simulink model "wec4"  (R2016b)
settings: Solver=ode4  StartTime=0  StopTime=1000  FixedStep=0.005  MaxStep=0.005  RelTol=1e-3  EnableMultiTasking=on
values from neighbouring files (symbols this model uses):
  arAdaptiveLawData = 1/2*zModelSimple.zModelPto.arFreq.*     zModelSimple.zModelPto.arMagnitude./     cos(zModelSimple.zModelPto.arPhase*pi/180+pi/2)    [IMPACT_Control.m]
  arAdaptiveLawDataX = 1/2*zModelSimpleX.zModelPto.arFreq.*         zModelSimpleX.zModelPto.arMagnitude./         cos(zModelSimpleX.zModelPto.arPhase*pi/180+pi/2)    [IMPACT_Control.m]
  arControllerRampGain = [0,0,1,1]    [IMPACT_Control.m]
  arControllerRampTime = [0 rStartRampTime rStartRampTime+rRampTimeLength 8000]    [IMPACT_Control.m]
  arEkfInitialisation = zeros(1,11)    [IMPACT_Control.m]
  arEkfInitialisationX = zeros(1,11)    [IMPACT_Control.m]
  arFrequency = zModelSimple.zModelPto.arFreq    [IMPACT_Control.m]
  arFrequencyRange = zModelSimple.zModelPto.arFreq    [IMPACT_Control.m]
  arFrequencyX = zModelSimpleX.zModelPto.arFreq    [IMPACT_Control.m]
  arImpedance = 1./zModelSimple.zModelPto.arMagnitude./zModelSimple.zModelPto.arFreq    [IMPACT_Control.m]
  arImpedanceX = 1./zModelSimpleX.zModelPto.arMagnitude./zModelSimpleX.zModelPto.arFreq    [IMPACT_Control.m]
  CentralPTOPreload = -1.6113e+07    (= -16113000)    [wecSimInputFile.m]
  F1 = [4.243 2.375 -12.243]    [wecSimInputFile.m]
  F2 = [4.243 -2.375 -12.243]    [wecSimInputFile.m]
  F3 = [-4.243 -2.375 -12.243]    [wecSimInputFile.m]
  F4 = [-4.243 2.375 -12.243]    [wecSimInputFile.m]
  FC = [0 0 -14]    [wecSimInputFile.m]
  iAdaptiveDamping = 0    [wec4IMPACT_Project.m]    (also in IMPACT_Control.m = handles.iAdaptiveDamping; wec1_IMPACT_Project.m; wec2_IMPACT_Project.m; wec3_IMPACT_Project.m)
  iControlType = 2    [wec4IMPACT_Project.m]    (also in IMPACT_Control.m = handles.iControlType; wec1_IMPACT_Project.m = 1; wec2_IMPACT_Project.m = 1; wec3_IMPACT_Project.m = 1)
  iPtoPositionConstraint = 1    [wec4IMPACT_Project.m]    (also in IMPACT_Control.m = handles.iPtoPositionConstraint; wec1_IMPACT_Project.m = 0; wec2_IMPACT_Project.m; wec3_IMPACT_Project.m)
  iSensorNoise = 0    [IMPACT_Control.m]
  m = m+1    (= 2)    [checkParamFile.m]
  PTOrotation = atan((T1(2)-F1(2))/(T1(1)-F1(1)))    [wecSimInputFile.m]
  rCogFloater = -8    [wec4_IMPACT_Model.m]    (also in paramInitial.m = get( handles.edit_rCogFloater, 'String' ); wec1_IMPACT_Model.m = -18; wec2_IMPACT_Model.m = -8.5; wec3_IMPACT_Model.m = -0.7)
  rCogSpar = -36.6    [wec4_IMPACT_Model.m]    (also in paramInitial.m = get( handles.edit_rCogSpar, 'String' ); wec3_IMPACT_Model.m = -21.3; wec3_IMPACT_Model2.m = -21.3)
  rDisplacementLimit = 10.000000    (= 10)    [wec4IMPACT_Project.m]    (also in IMPACT_Control.m = getValue(handles.edit_displacementLimit); wec1_IMPACT_Project.m; wec2_IMPACT_Project.m; wec3_IMPACT_Project.m = 3)
  rDisplacementLimitX = 10.000000    (= 10)    [wec4IMPACT_Project.m]    (also in IMPACT_Control.m = getValue(handles.edit_displacementLimitX); wec1_IMPACT_Project.m = 0; wec2_IMPACT_Project.m; wec3_IMPACT_Project.m = 0)
  rGainForAntiWIndUp = tfControllerDiscrete.rGain    [IMPACT_Control.m]
  rGainForAntiWIndUpX = tfControllerXDiscrete.rGain    [IMPACT_Control.m]
  rMaxForcePto = 300000000.000000    (= 300000000)    [wec4IMPACT_Project.m]    (also in IMPACT_Control.m = getValue(handles.edit_maxForcePto); wec1_IMPACT_Project.m = 1e+15; wec2_IMPACT_Project.m = 1e+15; wec3_IMPACT_Project.m = 1000000000)
  rMinForcePto = -300000000.000000    (= -300000000)    [wec4IMPACT_Project.m]    (also in IMPACT_Control.m = getValue(handles.edit_minForcePto); wec1_IMPACT_Project.m = -1e+15; wec2_IMPACT_Project.m = -1e+15; wec3_IMPACT_Project.m = -1000000000)
  rMooringX = 20000    [wec4_IMPACT_Model.m]    (also in paramInitial.m = get( handles.edit_rMooringX, 'String' ); wec3_IMPACT_Model.m = 10000; wec3_IMPACT_Model2.m = 10000)
  rMooringZ = 10000    [wec4_IMPACT_Model.m]    (also in paramInitial.m = get( handles.edit_rMooringZ, 'String' ); wec3_IMPACT_Model.m = 0; wec3_IMPACT_Model2.m = 0)
  rOutputSampleTime = 0.010000    (= 0.01)    [wec4IMPACT_Project.m]    (also in IMPACT_Control.m = getValue(handles.edit_outputSampleTime); wec1_IMPACT_Project.m; wec2_IMPACT_Project.m; wec3_IMPACT_Project.m)
  rPassiveDampingGain = -604830.000000    (= -604830)    [wec4IMPACT_Project.m]    (also in IMPACT_Control.m = getValue(handles.edit_gainPLD); wec1_IMPACT_Project.m = -214018.1537; wec2_IMPACT_Project.m = -1948070; wec3_IMPACT_Project.m = -519390)
  rPassiveDampingGainX = -278660.000000    (= -278660)    [wec4IMPACT_Project.m]    (also in IMPACT_Control.m = getValue(handles.edit_gainPLDX); wec1_IMPACT_Project.m = 0; wec2_IMPACT_Project.m = 0; wec3_IMPACT_Project.m = 0)
  rTetherPretension = 1.6113e+07    (= 16113000)    [wec4_IMPACT_Model.m]    (also in paramInitial.m = get( handles.edit_rTetherPretension, 'String' ); wec3_IMPACT_Model.m = 0; wec3_IMPACT_Model2.m = 0)
  rTetherSpring = 500000    [wec4_IMPACT_Model.m]    (also in paramInitial.m = get( handles.edit_rTetherSpring, 'String' ); wec3_IMPACT_Model.m = 0; wec3_IMPACT_Model2.m = 0)
  rUpperFrequencyLimit = EKFFloater.upperFreq    [IMPACT_Control.m]
  rXf = 4.243    [wec4AdditionalParams.m]
  rXs = 16.075    [wec4AdditionalParams.m]
  rYf = 2.375    [wec4AdditionalParams.m]
  rYs = 16.075    [wec4AdditionalParams.m]
  rZf = 4.243    [wec4AdditionalParams.m]
  rZs = 2.4350    (= 2.435)    [wec4AdditionalParams.m]
  rZTetherF = 6    [wec4AdditionalParams.m]
  rZTetherS = 2.4350    (= 2.435)    [wec4AdditionalParams.m]
  s = tf('s')    [wec4_IMPACT_Model.m]    (also in IMPACT_Control.m; wec1_IMPACT_Model.m; wec2_IMPACT_Model.m; wec3_IMPACT_Model.m)
  SidePTO1Preload = PreloadPTOCorner    (= 0)    [wecSimInputFile.m]
  SidePTO2Preload = PreloadPTOCorner    (= 0)    [wecSimInputFile.m]
  SidePTO3Preload = PreloadPTOCorner    (= 0)    [wecSimInputFile.m]
  SidePTO4Preload = PreloadPTOCorner    (= 0)    [wecSimInputFile.m]
  simu = simulationClass()    [wecSimInputFile.m]
  T1 = [16.075 16.075 -34.165]    [wecSimInputFile.m]
  T2 = [16.075 -16.075 -34.165]    [wecSimInputFile.m]
  T3 = [-16.075 -16.075 -34.165]    [wecSimInputFile.m]
  T4 = [-16.075 16.075 -34.165]    [wecSimInputFile.m]
  TC = [0 0 -34.165]    [wecSimInputFile.m]
  waves = waveClass('irregular')    [wecSimInputFile.m]
  Z = magPhaseToComplex(zModelTf)    [IMPACT_Control.m]
undefined symbols (not defined in the file or in its folder): arControllerDiscreteDen, arControllerDiscreteNum, arControllerDiscreteXDen, arControllerDiscreteXNum, arExcForceFloaterDen, arExcForceFloaterNum, arExcForceFloaterXDen, arExcForceFloaterXNum, arExcForceSparDen, arExcForceSparNum, arExcForceSparXDen, arExcForceSparXNum, arFexcFloaterDen, arFexcFloaterNum, arFexcFloaterXDen, arFexcFloaterXNum, arFexcSparDen, arFexcSparNum, arFexcSparXDen, arFexcSparXNum, Body, body, constraint, CTTime, deg, Elements, geometry, IRKB, kg, lenJ, mooring, N, pto, rAccelerationGainFloater, rAccelerationGainFloaterX, rAccelerationGainSpar, rAccelerationGainSparX, rad, rBuoyancyGainFloater, rBuoyancyGainFloaterX, rBuoyancyGainSpar, rBuoyancyGainSparX, rDampingGainFloater, rDampingGainFloaterX, rDampingGainSpar, rDampingGainSparX, Rigid, rMaxFocePto, wec4_float, wec4_reactor, WECSim_Lib, X, Y
libraries: nesl_utility x380, sm_lib x170, vrlib x91, simulink x12, WECSim_Lib x4
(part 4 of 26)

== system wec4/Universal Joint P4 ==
  Assignment : Assignment  DiagnosticForDimensions=Warning  IndexOptions=Index vector (dialog)  Indices=[4 5]  OutputSizes=1
  Assignment1 : Assignment  DiagnosticForDimensions=Warning  IndexOptions=Index vector (dialog)  Indices=[4 5]  OutputSizes=1
  Assignment2 : Assignment  DiagnosticForDimensions=Warning  IndexOptions=Index vector (dialog)  Indices=[4 5]  OutputSizes=1
  CONSTRAINT Universal Joint : sm_lib/Joints/Universal Joint  SenseConstraintForce=on  SenseConstraintForceX=off  SenseConstraintForceY=off  SenseConstraintForceZ=off  SenseConstraintTorque=on  SenseConstraintTorqueX=off  SenseConstraintTorqueY=off  SenseConstraintTorqueZ=off  SenseTotalForce=off  SenseTotalForceX=off  SenseTotalForceY=off  SenseTotalForceZ=off  SenseTotalTorque=off  SenseTotalTorqueX=off  SenseTotalTorqueY=off  SenseTotalTorqueZ=off  CompositeWrenchDir=BaseOnFollower  CompositeWrenchFrame=BaseFrame  RxEquilibriumPosition=0  RxEquilibriumPositionUnits=deg  RxSpringStiffness=0  RxSpringStiffnessUnits=N*m/deg  RxDampingCoefficient=0  RxDampingCoefficientUnits=N*m/(deg/s)  RxTorqueActuationMode=NoTorque  RxMotionActuationMode=ComputedMotion  RxSensePosition=on  RxSenseVelocity=on  RxSenseAcceleration=on  RxSenseTorqueForce=off  RxPositionTargetSpecify=off  RxPositionTargetPriority=High  RxPositionTargetValue=0  RxPositionTargetValueUnits=deg  RxVelocityTargetSpecify=off  RxVelocityTargetPriority=High  RxVelocityTargetValue=0  RxVelocityTargetValueUnits=deg/s  RyEquilibriumPosition=0  RyEquilibriumPositionUnits=deg  RySpringStiffness=0  RySpringStiffnessUnits=N*m/deg  RyDampingCoefficient=0  RyDampingCoefficientUnits=N*m/(deg/s)  RyTorqueActuationMode=NoTorque  RyMotionActuationMode=ComputedMotion  RySensePosition=on  RySenseVelocity=on  RySenseAcceleration=on  RySenseTorqueForce=off  RyPositionTargetSpecify=off  RyPositionTargetPriority=High  RyPositionTargetValue=0  RyPositionTargetValueUnits=deg  RyVelocityTargetSpecify=off  RyVelocityTargetPriority=High  RyVelocityTargetValue=0  RyVelocityTargetValueUnits=deg/s
  Constant : Constant  Value=[0 0 0 0 0 0]
  Constant1 : Constant  Value=[0 0 0 0 0 0]
  Constant2 : Constant  Value=[0 0 0 0 0 0]
  Mux{,2..4} (4 alike) : Mux  Inputs=2
  Mux1 : Mux
  PS-Simulink Converter{1..5,7,9,11} (8 alike) : nesl_utility/PS-Simulink Converter  PhysicalDomain=network_engine_domain  SubClassName=ps_output  LeftPortType=input  RightPortType=output  PseudoPeriodic=off  Frequencies=[]  Unit=1  AffineConversion=off
  Rigid Transform (Position) : sm_lib/Frames and Transforms/Rigid Transform  TranslationMethod=Cartesian  TranslationStandardOffset=0  TranslationLengthUnit=m  TranslationStandardAxis=+Z  TranslationCartesianOffset=constraint.initDisp.initLinDisp+constraint.loc  TranslationROffset=0  TranslationROffsetUnits=m  TranslationZOffset=0  TranslationZOffsetUnits=m  TranslationThetaOffset=0  TranslationThetaOffsetUnits=deg  RotationMethod=None  RotationAngleUnits=rad  RotationStandardAxis=+Y  RotationAngle=0  RotationArbitraryAxis=[0 1 0]  FollAlignAxisA=+X  BaseAlignAxisA=+Y  FollAlignAxisB=+Y  BaseAlignAxisB=+Z  RotationSequenceAxes=FollowerAxes  RotationSequence=XYX  RotationSequenceAngles=[0 0 0]  RotationSequenceAnglesUnits=deg  RotationMatrix=[1 0 0; 0 1 0; 0 0 1]
  Rigid Transform (Position)1 : sm_lib/Frames and Transforms/Rigid Transform  TranslationMethod=Cartesian  TranslationStandardOffset=0  TranslationLengthUnit=m  TranslationStandardAxis=+Z  TranslationCartesianOffset=constraint.initDisp.initLinDisp+constraint.loc  TranslationROffset=0  TranslationROffsetUnits=m  TranslationZOffset=0  TranslationZOffsetUnits=m  TranslationThetaOffset=0  TranslationThetaOffsetUnits=deg  RotationMethod=None  RotationAngleUnits=rad  RotationStandardAxis=+Y  RotationAngle=0  RotationArbitraryAxis=[0 1 0]  FollAlignAxisA=+X  BaseAlignAxisA=+Y  FollAlignAxisB=+Y  BaseAlignAxisB=+Z  RotationSequenceAxes=FollowerAxes  RotationSequence=XYX  RotationSequenceAngles=[0 0 0]  RotationSequenceAnglesUnits=deg  RotationMatrix=[1 0 0; 0 1 0; 0 0 1]
  Rigid Transform (Orientation) : sm_lib/Frames and Transforms/Rigid Transform  TranslationMethod=None  TranslationStandardOffset=0  TranslationLengthUnit=m  TranslationStandardAxis=+Z  TranslationCartesianOffset=constraint.loc  TranslationROffset=0  TranslationROffsetUnits=m  TranslationZOffset=0  TranslationZOffsetUnits=m  TranslationThetaOffset=0  TranslationThetaOffsetUnits=deg  RotationMethod=RotationMatrix  RotationAngleUnits=rad  RotationStandardAxis=+Y  RotationAngle=0  RotationArbitraryAxis=[0 1 0]  FollAlignAxisA=+X  BaseAlignAxisA=+Y  FollAlignAxisB=+Y  BaseAlignAxisB=+Z  RotationSequenceAxes=FollowerAxes  RotationSequence=XYX  RotationSequenceAngles=[0 0 0]  RotationSequenceAnglesUnits=deg  RotationMatrix=constraint.orientation.rotationMatrix
  Rigid Transform (Orientation)1 : sm_lib/Frames and Transforms/Rigid Transform  TranslationMethod=None  TranslationStandardOffset=0  TranslationLengthUnit=m  TranslationStandardAxis=+Z  TranslationCartesianOffset=constraint.loc  TranslationROffset=0  TranslationROffsetUnits=m  TranslationZOffset=0  TranslationZOffsetUnits=m  TranslationThetaOffset=0  TranslationThetaOffsetUnits=deg  RotationMethod=RotationMatrix  RotationAngleUnits=rad  RotationStandardAxis=+Y  RotationAngle=0  RotationArbitraryAxis=[0 1 0]  FollAlignAxisA=+X  BaseAlignAxisA=+Y  FollAlignAxisB=+Y  BaseAlignAxisB=+Z  RotationSequenceAxes=FollowerAxes  RotationSequence=XYX  RotationSequenceAngles=[0 0 0]  RotationSequenceAnglesUnits=deg  RotationMatrix=constraint.orientation.rotationMatrix
  output : ToWorkspace  VariableName=constraint10_out  SaveFormat=Structure With Time  SampleTime=-1
  F : PMIOPort  Port=1  Side=Right
  B : PMIOPort  Port=2  Side=Left
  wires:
  PS-Simulink Converter4/1 -> Mux/2
  PS-Simulink Converter3/1 -> Mux/1
  Mux3/1 -> Assignment1/2
  Mux4/1 -> Assignment/2
  Constant/1 -> Assignment/1
  Constant1/1 -> Assignment1/1
  Constant2/1 -> Assignment2/1
  Assignment2/1 -> Mux1/3  "acceleration"
  Assignment1/1 -> Mux1/2  "velocity"
  Assignment/1 -> Mux1/1  "position"
  Mux/1 -> Mux1/4  "Constraint Forces"
  Mux1/1 -> output/1
  PS-Simulink Converter5/1 -> Mux2/2
  Mux2/1 -> Assignment2/2
  PS-Simulink Converter2/1 -> Mux3/2
  PS-Simulink Converter9/1 -> Mux3/1
  PS-Simulink Converter11/1 -> Mux4/2
  PS-Simulink Converter1/1 -> Mux4/1
  PS-Simulink Converter7/1 -> Mux2/1
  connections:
  Rigid Transform (Position)1/LConn1 -- F/RConn1
  Rigid Transform (Position)1/RConn1 -- Rigid Transform (Orientation)1/LConn1
  Rigid Transform (Orientation)/RConn1 -- CONSTRAINT Universal Joint/LConn1
  Rigid Transform (Position)/RConn1 -- Rigid Transform (Orientation)/LConn1
  Rigid Transform (Position)/LConn1 -- B/RConn1
  CONSTRAINT Universal Joint/RConn8 -- PS-Simulink Converter3/LConn1
  PS-Simulink Converter4/LConn1 -- CONSTRAINT Universal Joint/RConn9
  PS-Simulink Converter1/LConn1 -- CONSTRAINT Universal Joint/RConn2
  PS-Simulink Converter11/LConn1 -- CONSTRAINT Universal Joint/RConn5
  PS-Simulink Converter9/LConn1 -- CONSTRAINT Universal Joint/RConn3
  PS-Simulink Converter7/LConn1 -- CONSTRAINT Universal Joint/RConn4
  PS-Simulink Converter2/LConn1 -- CONSTRAINT Universal Joint/RConn6
  PS-Simulink Converter5/LConn1 -- CONSTRAINT Universal Joint/RConn7
  CONSTRAINT Universal Joint/RConn1 -- Rigid Transform (Orientation)1/RConn1

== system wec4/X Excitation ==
  PTO force X : Inport
  Force estimation Floater X : Subsystem
  Force estimation Spar X : Subsystem
  Gain12 : Gain  Gain=rMooringX
  Gain3 : Gain  Gain=-1
  Rate Transition3 : RateTransition  OutPortSampleTimeMultiple=0.01  OutPortSampleTime=rKalmanFilterSampleTime
  Rate Transition4 : RateTransition  OutPortSampleTimeMultiple=0.01  OutPortSampleTime=rKalmanFilterSampleTime
  Scope{11..14} (4 alike) : Scope
  Selector{7..12,22} (7 alike) : Selector  InputPortWidth=6  IndexOptions=Index vector (dialog)  Indices=1  OutputSizes=1
  Sum11 : Sum
  Sum4 : Sum  Inputs=|++
  Sum5 : Sum  Inputs=|+-
  To Workspace11 : ToWorkspace  VariableName=arForceXFloater  SampleTime=rOutputSampleTime
  To Workspace5 : ToWorkspace  VariableName=arExcitationForceSparX  SampleTime=rOutputSampleTime
  To Workspace6 : ToWorkspace  VariableName=arExcitationForceFloaterX  SampleTime=rOutputSampleTime
  floaterExcitation : Outport
  SparExcitation : Outport  Port=2
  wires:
  Sum4/1 -> Scope14/1
  Selector8/1 -> Force estimation Floater X/3(Position)
  Selector7/1 -> Force estimation Floater X/2(Velocity)
  [acc1] -> Selector9/1
  [acc2] -> Selector12/1
  Sum5/1 -> Scope11/1
  Gain3/1 -> Sum11/1
  [vel1] -> Selector7/1
  Selector10/1 -> Force estimation Spar X/2(Velocity)
  [disp1] -> Selector8/1
  Selector12/1 -> Force estimation Spar X/1(Acceleration)
  Selector11/1 -> Force estimation Spar X/3(Position)
  Selector9/1 -> Force estimation Floater X/1(Acceleration)
  Force estimation Spar X/1(excForce) -> Rate Transition4/1
  Rate Transition3/1 -> To Workspace6/1, floaterExcitation/1, Scope13/1, Sum4/1, Sum5/1
  [disp2] -> Selector11/1
  Force estimation Floater X/1(excForce) -> Rate Transition3/1
  [vel2] -> Selector10/1
  PTO force X/1 -> Force estimation Floater X/4(PTO Force), Gain3/1, To Workspace11/1
  [disp2] -> Selector22/1
  Selector22/1 -> Gain12/1
  Gain12/1 -> Sum11/2
  Sum11/1 -> Force estimation Spar X/4(PTO Force)
  Rate Transition4/1 -> To Workspace5/1, SparExcitation/1, Sum4/2, Sum5/2, Scope12/1

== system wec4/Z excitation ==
  PTO force Z : Inport
  Constant2 : Constant  Value=rCogSpar
  "Force estimation Floater " : Subsystem
  Force estimation Spar : Subsystem
  Gain : Gain  Gain=-1
  Gain12 : Gain  Gain=rMooringZ
  Rate Transition1 : RateTransition  OutPortSampleTimeMultiple=0.01  OutPortSampleTime=rKalmanFilterSampleTime
  Rate Transition2 : RateTransition  OutPortSampleTimeMultiple=0.01  OutPortSampleTime=rKalmanFilterSampleTime
  Selector{1..6,22} (7 alike) : Selector  InputPortWidth=6  IndexOptions=Index vector (dialog)  Indices=3  OutputSizes=1
  Sum11 : Sum
  Sum20 : Sum  Inputs=+-
  To Workspace4 : ToWorkspace  VariableName=arExcitationForceSpar  SampleTime=rOutputSampleTime
  To Workspace7 : ToWorkspace  VariableName=arExcitationForceFloater  SampleTime=rOutputSampleTime
  floaterExcitation : Outport
  SparExcitation : Outport  Port=2
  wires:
  Selector4/1 -> Force estimation Spar/2(Velocity)
  Rate Transition2/1 -> SparExcitation/1, To Workspace4/1
  Selector5/1 -> Force estimation Spar/3(Position)
  Gain/1 -> Sum11/1
  "Force estimation Floater "/1(excForce) -> Rate Transition1/1
  [acc1] -> Selector3/1
  Force estimation Spar/1(excForce) -> Rate Transition2/1
  [vel1] -> Selector1/1
  Rate Transition1/1 -> floaterExcitation/1, To Workspace7/1
  PTO force Z/1 -> "Force estimation Floater "/4(PTO Force), Gain/1
  Selector6/1 -> Force estimation Spar/1(Acceleration)
  [acc2] -> Selector6/1
  [vel2] -> Selector4/1
  [disp1] -> Selector2/1
  [disp2] -> Selector5/1
  Constant2/1 -> Sum20/2
  [disp2] -> Selector22/1
  Gain12/1 -> Sum11/2
  Sum20/1 -> Gain12/1
  Sum11/1 -> Force estimation Spar/4(PTO Force)
  Selector22/1 -> Sum20/1
  Selector3/1 -> "Force estimation Floater "/1(Acceleration)
  Selector1/1 -> "Force estimation Floater "/2(Velocity)
  Selector2/1 -> "Force estimation Floater "/3(Position)

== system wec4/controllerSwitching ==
  ovtForceDemand1 : Inport
  ovtForceDemand2 : Inport  Port=2
  ovtForceDemand3 : Inport  Port=3
  ovtForceDemand4 : Inport  Port=4
  linearDampingForce1 : Inport  Port=5
  linearDampingForce2 : Inport  Port=6
  linearDampingForce3 : Inport  Port=7
  linearDampingForce4 : Inport  Port=8
  Constant2 : Constant  Value=iControlType
  Mux1 : Mux
  Mux11 : Mux
  Saturation : Saturate  Commented=through  UpperLimit=rMaxForcePto  LowerLimit=-rMaxFocePto
  Switch1 : Switch  Threshold=2
  forceDemand : Outport
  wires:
  linearDampingForce1/1 -> Mux1/1
  linearDampingForce2/1 -> Mux1/2
  linearDampingForce3/1 -> Mux1/3
  linearDampingForce4/1 -> Mux1/4
  Constant2/1 -> Switch1/2
  Mux11/1 -> Switch1/3
  Mux1/1 -> Switch1/1
  Switch1/1 -> Saturation/1
  Saturation/1 -> forceDemand/1
  ovtForceDemand1/1 -> Mux11/1
  ovtForceDemand2/1 -> Mux11/2
  ovtForceDemand3/1 -> Mux11/3
  ovtForceDemand4/1 -> Mux11/4

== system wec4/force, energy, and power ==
  Gain1 : Gain  Gain=-1
  Integrator : Integrator
  Mux1 : Mux
  Product{,1..3} (4 alike) : Product
  Scope : Scope
  Scope6 : Scope
  Scope7 : Scope
  Sum : Sum  Inputs=++++
  To Workspace1 : ToWorkspace  VariableName=arPtoForceOutput  SampleTime=rOutputSampleTime
  To Workspace2 : ToWorkspace  VariableName=arWecPower  SampleTime=rOutputSampleTime
  To Workspace3 : ToWorkspace  VariableName=arWecEnergy  SampleTime=rOutputSampleTime
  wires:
  Mux1/1 -> To Workspace1/1, Scope/1
  [ptoForce4] -> Product3/2, Mux1/4
  [ptoForce3] -> Product2/1, Mux1/3
  [ptoForce2] -> Product1/1, Mux1/2
  [ptoForce1] -> Product/1, Mux1/1
  [ptoSpd1] -> Product/2
  [ptoSpd2] -> Product1/2
  [ptoSpd3] -> Product2/2
  [ptoSpd4] -> Product3/1
  Product/1 -> Sum/1
  Product1/1 -> Sum/2
  Product2/1 -> Sum/3
  Product3/1 -> Sum/4
  Sum/1 -> Gain1/1
  Integrator/1 -> Scope6/1, To Workspace3/1
  Gain1/1 -> Integrator/1, Scope7/1, To Workspace2/1

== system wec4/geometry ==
  Constant : Constant  Value="sqrt( (F1(1)-T1(1))^2 + (F1(2)-T1(2))^2 + (F1(3)-T1(3))^2  )"
  Demux{1..3,8} (4 alike) : Demux
  Divide : Product  Inputs=/*
  Geometry1 : Subsystem
  Math Function : Math  Operator=square
  Math Function1 : Math  Operator=square
  Mux{1,12,14,24} (4 alike) : Mux
  Sqrt : Sqrt
  Subsystem4 : Subsystem
  Sum : Sum  Inputs=|++
  Sum1 : Sum  Inputs=|++
  "Terminator2 " : Terminator
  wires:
  Demux8/4 -> [kappa4]
  Demux2/1 -> [beta1]
  Demux2/3 -> [beta3]
  Demux3/3 -> [gamma3]
  Demux8/1 -> [kappa1]
  Demux8/3 -> [kappa3]
  Mux12/1 -> Subsystem4/2(mus)
  Mux14/1 -> [zetas], Math Function/1, Subsystem4/1(Zetas)
  Geometry1/1(zeta1) -> Mux14/1
  Geometry1/2(zeta2) -> Mux14/2
  Geometry1/3(zeta3) -> Mux14/3
  Geometry1/4(zeta4) -> Mux14/4
  Geometry1/5(mu1) -> Mux12/1
  Geometry1/6(mu2) -> Mux12/2
  Geometry1/7(mu3) -> Mux12/3
  Geometry1/8(mu4) -> Mux12/4
  Mux24/1 -> Math Function1/1, Subsystem4/3(etas), [etas]
  Geometry1/9(eta1) -> Mux24/1
  Geometry1/10(eta2) -> Mux24/2
  Geometry1/11(eta3) -> Mux24/3
  Geometry1/12(eta4) -> Mux24/4
  Demux3/1 -> [gamma1]
  Demux3/4 -> [gamma4]
  Subsystem4/2(betas) -> Demux2/1
  Demux2/4 -> [beta4]
  Demux2/2 -> [beta2]
  Demux3/2 -> [gamma2]
  Demux8/2 -> [kappa2]
  Subsystem4/4(alphas) -> Demux8/1
  Math Function/1 -> Sum/1
  Math Function1/1 -> Sum/2
  Sum/1 -> Sqrt/1
  [ptoDis1] -> Mux1/1
  [ptoDis2] -> Mux1/2
  [ptoDis3] -> Mux1/3
  [ptoDis4] -> Mux1/4
  Mux1/1 -> Sum1/2
  Sqrt/1 -> Divide/2
  Divide/1 -> Demux1/1
  Constant/1 -> Sum1/1
  Sum1/1 -> Divide/1
  Demux1/1 -> [cosAlpha1]
  Demux1/2 -> [cosAlpha2]
  Demux1/3 -> [cosAlpha3]
  Demux1/4 -> [cosAlpha4]
  Subsystem4/3(deltas) -> "Terminator2 "/1
  Subsystem4/1(gammas) -> Demux3/1

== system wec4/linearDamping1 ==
  ekfFrequencyZ : Inport
  ekfFrequencyX : Inport  Port=2
  Rel. vel X : Inport  Port=3
  Rel. vel. Z : Inport  Port=4
  Clock1 : Clock
  Constant3 : Constant  Value=iAdaptiveDamping
  Constant4 : Constant  Value=rPassiveDampingGain
  Constant5 : Constant  Value=iAdaptiveDamping
  Constant6 : Constant  Value=rPassiveDampingGainX
  Gain1 : Gain  Gain=-1
  Gain3 : Gain  Gain=-1
  Product{1..3,11} (4 alike) : Product
  Ramp gain2 : Lookup_n-D  NumberOfTableDimensions=1  BreakpointsForDimension1=arControllerRampTime  Table=arControllerRampGain  InternalRulePriority=Speed  RndMeth=Simplest
  Switch1 : Switch  Criteria=u2 > Threshold
  Switch2 : Switch  Criteria=u2 > Threshold
  Trnasformation X-Z into PTO forces : Subsystem
  adaptiveLaw1 : Lookup_n-D  NumberOfTableDimensions=1  BreakpointsForDimension1=arFrequencyX  Table=arImpedanceX  InternalRulePriority=Speed  RndMeth=Simplest
  adaptiveLaw2 : Lookup_n-D  NumberOfTableDimensions=1  BreakpointsForDimension1=arFrequency  Table=arImpedance  InternalRulePriority=Speed  RndMeth=Simplest
  forceDemand1 : Outport
  forceDemand2 : Outport  Port=2
  forceDemand3 : Outport  Port=3
  forceDemand4 : Outport  Port=4
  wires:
  adaptiveLaw2/1 -> Gain3/1
  ekfFrequencyZ/1 -> adaptiveLaw2/1
  adaptiveLaw1/1 -> Gain1/1
  ekfFrequencyX/1 -> adaptiveLaw1/1
  Constant3/1 -> Switch2/2
  Gain3/1 -> Switch2/1  "K_z"
  Constant4/1 -> Switch2/3
  Constant5/1 -> Switch1/2
  Gain1/1 -> Switch1/1  "K_x"
  Constant6/1 -> Switch1/3
  Switch2/1 -> Product2/1  "Impedance Z"
  Switch1/1 -> Product1/2  "Impedance X"
  Clock1/1 -> Ramp gain2/1
  Ramp gain2/1 -> Product3/1, Product11/2
  Product3/1 -> forceDemand2/1, forceDemand1/1  "F1"
  Trnasformation X-Z into PTO forces/1(Force PTOs 3-4) -> Product11/1
  Product11/1 -> forceDemand4/1, forceDemand3/1
  Trnasformation X-Z into PTO forces/2(Force PTOs 1-2) -> Product3/2
  Rel. vel. Z/1 -> Product2/2
  Rel. vel X/1 -> Product1/1
  Product1/1 -> Trnasformation X-Z into PTO forces/1(Force X)
  Product2/1 -> Trnasformation X-Z into PTO forces/2(Force Z)

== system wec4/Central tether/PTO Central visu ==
  note: 1) Add Subsystem or Model blocks as valid variant choices. 2) You cannot connect blocks at this level. At simulation, connectivity is automatically determined, based on the active variant and port name matching.
  Hydrodynamic Body : Subsystem  VariantControl=sv_b3_hydroBody
  Non-Hydro Body : Subsystem  VariantControl=sv_b3_nonHydroBody
  Conn : PMIOPort  Port=1  Side=Right

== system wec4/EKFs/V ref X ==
  phiOut : Inport
  ekfFrequency : Inport  Port=2
  ekfAmplitude : Inport  Port=3
  Constraint : Subsystem
  Divide4 : Product  Inputs=**
  Gain1 : Gain
  Product1 : Product
  Scope2 : Scope
  Transfer Fcn : TransferFcn  Denominator=[0.05 1]
  adaptiveLaw : Lookup_n-D  NumberOfTableDimensions=1  BreakpointsForDimension1=arFrequencyRange  Table=arAdaptiveLawDataX  InternalRulePriority=Speed  RndMeth=Simplest
  adaptiveLaw1 : Lookup_n-D  NumberOfTableDimensions=1  BreakpointsForDimension1=arFrequencyRange  Table=arFrequencyRange./arFrequencyRange  InternalRulePriority=Speed  RndMeth=Simplest
  referenceVelocity : Outport
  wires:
  Transfer Fcn/1 -> Product1/2
  Product1/1 -> Scope2/1, Divide4/1
  ekfAmplitude/1 -> Constraint/2(Amp)
  phiOut/1 -> Transfer Fcn/1
  ekfFrequency/1 -> adaptiveLaw/1, adaptiveLaw1/1, Constraint/3(ekfFrequency)
  Divide4/1 -> referenceVelocity/1
  adaptiveLaw/1 -> Gain1/1
  Gain1/1 -> Constraint/1(1/2B)
  Constraint/1(referenceVelocity) -> Product1/1
  adaptiveLaw1/1 -> Divide4/2

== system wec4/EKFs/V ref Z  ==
  phiOut : Inport
  ekfFrequency : Inport  Port=2
  ekfAmplitude : Inport  Port=3
  Constraint : Subsystem
  Divide4 : Product  Inputs=**
  Gain1 : Gain
  Product1 : Product
  Scope2 : Scope
  Transfer Fcn : TransferFcn  Denominator=[0.05 1]
  adaptiveLaw : Lookup_n-D  NumberOfTableDimensions=1  BreakpointsForDimension1=arFrequencyRange  Table=arAdaptiveLawData  InternalRulePriority=Speed  RndMeth=Simplest
  adaptiveLaw1 : Lookup_n-D  NumberOfTableDimensions=1  BreakpointsForDimension1=arFrequencyRange  Table=arFrequencyRange./arFrequencyRange  InternalRulePriority=Speed  RndMeth=Simplest
  referenceVelocity : Outport
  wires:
  Constraint/1(referenceVelocity) -> Product1/1
  Gain1/1 -> Constraint/1(1/2B)
  adaptiveLaw/1 -> Gain1/1
  Divide4/1 -> referenceVelocity/1
  ekfFrequency/1 -> adaptiveLaw1/1, Constraint/3(ekfFrequency), adaptiveLaw/1
  phiOut/1 -> Transfer Fcn/1
  ekfAmplitude/1 -> Constraint/2(Amp)
  Product1/1 -> Scope2/1, Divide4/1
  Transfer Fcn/1 -> Product1/2
  adaptiveLaw1/1 -> Divide4/2

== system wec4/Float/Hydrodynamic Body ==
  Additional Linear Damping Force Calculation : Subsystem
  B2B Subsystem : Subsystem  Variant=on
  Bus Creator : BusCreator  Inputs=6
  Bus Creator1 : BusCreator  Inputs=3
  Bus Selector1 : BusSelector  OutputSignals=F_Excitation,F_RadiationDamping,F_AddedMass,F_Restoring,F_MorrisonAndViscous,F_LinearDamping
  Bus Selector2 : BusSelector  OutputSignals=disp,vel,acc
  Hydrostatic Restoring Force Calculation : Subsystem
  Morrison Element and ViscousDampingForceCalculation : Subsystem
  Nonlinear Wave Elevation : Subsystem  TreatAsAtomicUnit=on  SystemSampleTime=simu.dtNL
  Structure : Subsystem
  Sum : Sum  Inputs=+-----
  To Workspace : ToWorkspace  VariableName=body1_out  SaveFormat=Structure With Time  SampleTime=-1
  Wave Diffraction and Excitation Force Calculation : Subsystem
  Wave Radiation Forces Calculation : Subsystem
  Conn : PMIOPort  Port=1  Side=Right
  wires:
  Additional Linear Damping Force Calculation/1(F_LinearDamping) -> Bus Creator/6
  Bus Creator/1 -> Bus Selector1/1, Bus Creator1/3  "BUS(7): Forces"
  Bus Selector2/1 -> [disp1]  "<disp>"
  Bus Selector2/3 -> [acc1]  "<acc>"
  Bus Selector2/2 -> [vel1]  "<vel>"
  Structure/1(Response) -> Bus Creator1/1, Bus Selector2/1
  Sum/1 -> Bus Creator1/2, Structure/1(Total Force)  "F_Total"
  Bus Creator1/1 -> To Workspace/1
  Bus Selector1/4 -> Sum/4  "<F_Restoring>"
  Bus Selector1/3 -> Sum/3  "<F_AddedMass>"
  Bus Selector1/5 -> Sum/5  "<F_MorrisonAndViscous>"
  Bus Selector1/2 -> Sum/2  "<F_RadiationDamping>"
  Bus Selector1/1 -> [Fex1], Sum/1  "<F_Excitation>"
  Bus Selector1/6 -> Sum/6  "<F_LinearDamping>"
  [acc1] -> B2B Subsystem/2(acc_in), Morrison Element and ViscousDampingForceCalculation/2(Acceleration)
  [vel1] -> Morrison Element and ViscousDampingForceCalculation/3(Velocity), Additional Linear Damping Force Calculation/1(Velocity), B2B Subsystem/1(vel_in)
  B2B Subsystem/2(acc) -> Wave Radiation Forces Calculation/2(Acceleration)
  B2B Subsystem/1(vel) -> Wave Radiation Forces Calculation/1(Velocity)
  [disp1] -> Hydrostatic Restoring Force Calculation/1(Displacement), Morrison Element and ViscousDampingForceCalculation/1(Displacement), Nonlinear Wave Elevation/1(Displacement), Wave Diffraction and Excitation Force Calculation/2(Displacement)
  Nonlinear Wave Elevation/1(Wave Elevation) -> Wave Diffraction and Excitation Force Calculation/3(WaveElv), Hydrostatic Restoring Force Calculation/2(Wave Elv)
  Hydrostatic Restoring Force Calculation/1(F_Restoring) -> Bus Creator/4
  Wave Radiation Forces Calculation/1(F_RadiationDamping) -> Bus Creator/2
  Wave Diffraction and Excitation Force Calculation/1(F_Excitation) -> Bus Creator/1
  Wave Radiation Forces Calculation/2(F_AddedMass) -> Bus Creator/3
  [Clock] -> Nonlinear Wave Elevation/2(Time), Wave Diffraction and Excitation Force Calculation/1(Time), Morrison Element and ViscousDampingForceCalculation/4(Time), Wave Radiation Forces Calculation/3(Time)
  Morrison Element and ViscousDampingForceCalculation/1(F_MorrisonAndViscous) -> Bus Creator/5
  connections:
  Conn/RConn1 -- Structure/RConn1

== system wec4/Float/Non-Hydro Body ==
  Bus Creator : BusCreator  Inputs=6
  Bus Creator1 : BusCreator  Inputs=3
  Bus Selector1 : BusSelector  OutputSignals=F_Excitation,F_RadiationDamping,F_AddedMass,F_Restoring,F_MorrisonAndViscous,F_LinearDamping
  Constant{,1..3,5} (5 alike) : Constant  Value=[0 0 0 0 0 0]
  Structure : Subsystem
  Sum : Sum  Inputs=+-----
  To Workspace : ToWorkspace  VariableName=body1_out  SaveFormat=Structure With Time  SampleTime=-1
  Weight and Buoyancy : Subsystem
  Conn : PMIOPort  Port=1  Side=Right
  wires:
  Bus Creator/1 -> Bus Creator1/3, Bus Selector1/1  "BUS(7): Forces"
  Structure/1(Response) -> Bus Creator1/1
  Sum/1 -> Bus Creator1/2, Structure/1(Total Force)  "F_Total"
  Bus Creator1/1 -> To Workspace/1
  Bus Selector1/4 -> Sum/4  "<F_Restoring>"
  Bus Selector1/3 -> Sum/3  "<F_AddedMass>"
  Bus Selector1/5 -> Sum/5  "<F_MorrisonAndViscous>"
  Bus Selector1/2 -> Sum/2  "<F_RadiationDamping>"
  Bus Selector1/1 -> Sum/1  "<F_Excitation>"
  Bus Selector1/6 -> Sum/6  "<F_LinearDamping>"
  Constant5/1 -> Bus Creator/6  "F_LinearDamping"
  Constant3/1 -> Bus Creator/5  "F_MorrisonAndViscous"
  Constant2/1 -> Bus Creator/3  "F_AddedMass"
  Constant1/1 -> Bus Creator/2  "F_RadiationDamping"
  Constant/1 -> Bus Creator/1  "F_Excitation"
  Weight and Buoyancy/1(Out1) -> Bus Creator/4  "F_Restoring"
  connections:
  Conn/RConn1 -- Structure/RConn1

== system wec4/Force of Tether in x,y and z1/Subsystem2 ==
  Constant1 : Constant  Value=rZTetherF
  Constant2 : Constant  Value=rZTetherS
  Constant3 : Constant  Value=rZTetherF
  Constant5 : Constant  Value=rZTetherS
  Gain : Gain  Gain=-1
  Gain1 : Gain  Gain=-1
  Product{,1..7} (8 alike) : Product
  Selector17 : Selector  InputPortWidth=6  IndexOptions=Index vector (dialog)  Indices=5  OutputSizes=1
  Selector18 : Selector  InputPortWidth=6  IndexOptions=Index vector (dialog)  Indices=4  OutputSizes=1
  Selector20 : Selector  InputPortWidth=6  IndexOptions=Index vector (dialog)  Indices=4  OutputSizes=1
  Selector21 : Selector  InputPortWidth=6  IndexOptions=Index vector (dialog)  Indices=5  OutputSizes=1
  Subsystem1 : Subsystem
  Sum : Sum  Inputs=|++
  Sum1 : Sum  Inputs=|++
  Sum2 : Sum  Inputs=|++
  Sum4 : Sum  Inputs=|--
  Sum5 : Sum  Inputs=--|
  Sum6 : Sum  Inputs=++|
  Trigonometric Function{,1,6..7} (4 alike) : Trigonometry
  Trigonometric Function{2..5} (4 alike) : Trigonometry  Operator=cos
  x_total : Outport
  y_total : Outport  Port=2
  z_total : Outport  Port=3
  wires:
  [disp1] -> Gain1/1
  [disp2] -> Gain/1
  Selector17/1 -> Trigonometric Function2/1, Trigonometric Function/1  "Phi"
  Trigonometric Function/1 -> Product/1
  Constant1/1 -> Product/2
  Constant2/1 -> Product1/1
  Trigonometric Function1/1 -> Product1/2
  Product/1 -> Sum/1
  Product1/1 -> Sum/2
  Sum/1 -> Sum1/1
  Subsystem1/1(x_r) -> Sum1/2
  Sum1/1 -> x_total/1
  Constant3/1 -> Product2/2
  Trigonometric Function2/1 -> Product2/1
  Product2/1 -> Product7/2, Product3/1  "z_f_phi"
  Selector18/1 -> Trigonometric Function7/1, Trigonometric Function3/1  "theta"
  Trigonometric Function3/1 -> Product3/2
  Sum2/1 -> z_total/1
  Subsystem1/3(z_r) -> Sum2/2
  Sum4/1 -> Sum2/1
  Constant5/1 -> Product4/2
  Trigonometric Function4/1 -> Product4/1
  Product4/1 -> Product6/2, Product5/1  "z_s_phi"
  Selector21/1 -> Trigonometric Function1/1, Trigonometric Function4/1  "Phi"
  Trigonometric Function5/1 -> Product5/2
  Product5/1 -> Sum4/2
  Product7/1 -> Sum5/1
  Product6/1 -> Sum5/2
  Sum5/1 -> Sum6/2
  Sum6/1 -> y_total/1
  Subsystem1/2(y_r) -> Sum6/1
  Product3/1 -> Sum4/1
  Selector20/1 -> Trigonometric Function5/1, Trigonometric Function6/1  "theta"
  Trigonometric Function6/1 -> Product6/1
  Trigonometric Function7/1 -> Product7/1
  Gain/1 -> Selector20/1, Selector21/1
  Gain1/1 -> Selector18/1, Selector17/1

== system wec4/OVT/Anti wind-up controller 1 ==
  error : Inport
  Add : Sum
  Add1 : Sum
  Add2 : Sum  Inputs=+-
  Clock3 : Clock
  Gain : Gain  Gain=rGainForAntiWIndUp
  Gain2 : Gain  Gain=1/rGainForAntiWIndUp
  Product : Product
  Ramp gain : Lookup_n-D  NumberOfTableDimensions=1  BreakpointsForDimension1=arControllerRampTime  Table=arControllerRampGain  InternalRulePriority=Speed  RndMeth=Simplest
  Saturation : Saturate  UpperLimit=rMaxForcePto  LowerLimit=rMinForcePto
  Transfer Fcn : TransferFcn  Numerator=arControllerDiscreteNum  Denominator=arControllerDiscreteDen
  Unit Delay : UnitDelay  SampleTime=0.01
  Unit Delay1 : UnitDelay  SampleTime=0.01
  forceDemand1 : Outport
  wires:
  Add/1 -> Saturation/1, Add2/2
  Gain/1 -> Add/2
  Unit Delay/1 -> Add1/2
  Gain2/1 -> Unit Delay1/1
  Add2/1 -> Gain2/1
  Add1/1 -> Transfer Fcn/1
  Transfer Fcn/1 -> Add/1
  Clock3/1 -> Ramp gain/1
  Ramp gain/1 -> Product/1
  Product/1 -> Add1/1
  Unit Delay1/1 -> Product/2
  error/1 -> Gain/1, Unit Delay/1
  Saturation/1 -> forceDemand1/1, Add2/1

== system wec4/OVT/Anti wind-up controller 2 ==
  error : Inport
  Add : Sum
  Add1 : Sum
  Add2 : Sum  Inputs=+-
  Clock3 : Clock
  Gain : Gain  Gain=rGainForAntiWIndUpX
  Gain2 : Gain  Gain=1/rGainForAntiWIndUpX
  Product : Product
  Ramp gain : Lookup_n-D  NumberOfTableDimensions=1  BreakpointsForDimension1=arControllerRampTime  Table=arControllerRampGain  InternalRulePriority=Speed  RndMeth=Simplest
  Saturation : Saturate  UpperLimit=rMaxForcePto  LowerLimit=rMinForcePto
  Transfer Fcn : TransferFcn  Numerator=arControllerDiscreteXNum  Denominator=arControllerDiscreteXDen
  Unit Delay : UnitDelay  SampleTime=0.01
  Unit Delay1 : UnitDelay  SampleTime=0.01
  forceDemand1 : Outport
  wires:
  Saturation/1 -> forceDemand1/1, Add2/1
  error/1 -> Unit Delay/1, Gain/1
  Unit Delay1/1 -> Product/2
  Product/1 -> Add1/1
  Ramp gain/1 -> Product/1
  Clock3/1 -> Ramp gain/1
  Transfer Fcn/1 -> Add/1
  Add1/1 -> Transfer Fcn/1
  Add2/1 -> Gain2/1
  Gain2/1 -> Unit Delay1/1
  Unit Delay/1 -> Add1/2
  Gain/1 -> Add/2
  Add/1 -> Add2/2, Saturation/1

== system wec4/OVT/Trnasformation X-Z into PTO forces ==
  Force X : Inport
  Force Z : Inport  Port=2
  Constant{,1..3} (4 alike) : Constant  Value=2
  Divide : Product  Inputs=/*
  Divide1 : Product  Inputs=/*
  Product{1..2,4..5,8..10,22} (8 alike) : Product
  Product{6..7,23..24} (4 alike) : Product  Inputs=3
  Sum10 : Sum  Inputs=|++
  Sum2 : Sum  Inputs=|+-
  Sum3 : Sum  Inputs=|++
  Sum4 : Sum  Inputs=|++
  Trigonometric Function{,1,8..9} (4 alike) : Trigonometry  Operator=cos
  Trigonometric Function{2..3,10..11} (4 alike) : Trigonometry
  Force PTOs 3-4 : Outport
  Force PTOs 1-2 : Outport  Port=2
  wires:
  [beta1] -> Trigonometric Function/1
  [beta3] -> Trigonometric Function1/1
  Divide/1 -> Force PTOs 1-2/1  "F1"
  Sum3/1 -> Divide/1
  Sum2/1 -> Divide/2
  Product7/1 -> Sum3/2
  Product6/1 -> Sum3/1
  Product4/1 -> Sum2/2
  Product5/1 -> Sum2/1
  Constant1/1 -> Product7/3
  Constant/1 -> Product6/3
  Trigonometric Function3/1 -> Product7/1  "sinLambda1"
  Trigonometric Function2/1 -> Product4/1, Product6/2  "sinLambda3"
  Product2/1 -> Product7/2, Product5/1  "cosLambda3"
  Trigonometric Function1/1 -> Product2/2
  [gamma3] -> Trigonometric Function2/1
  Product1/1 -> Product6/1  "cosLambda1"
  Trigonometric Function/1 -> Product1/2
  [gamma1] -> Trigonometric Function3/1
  Force Z/1 -> Product5/2, Product22/2
  Force X/1 -> Product4/2, Product10/2
  [beta3] -> Trigonometric Function8/1
  [beta1] -> Trigonometric Function9/1
  Sum10/1 -> Divide1/1
  Sum4/1 -> Divide1/2
  Product24/1 -> Sum10/2
  Product23/1 -> Sum10/1
  Product10/1 -> Sum4/2
  Product22/1 -> Sum4/1
  Constant3/1 -> Product24/3
  Constant2/1 -> Product23/3
  Trigonometric Function11/1 -> Product24/1  "sinLambda3"
  Trigonometric Function10/1 -> Product23/2, Product10/1  "sinLambda1"
  Product9/1 -> Product22/1, Product24/2  "cosLambda1"
  Trigonometric Function9/1 -> Product9/2
  [gamma1] -> Trigonometric Function10/1
  [cosAlpha3] -> Product8/1, Product2/1
  Product8/1 -> Product23/1  "cosLambda3"
  Trigonometric Function8/1 -> Product8/2
  [gamma3] -> Trigonometric Function11/1
  [cosAlpha1] -> Product9/1, Product1/1
  Divide1/1 -> Force PTOs 3-4/1  "F3"

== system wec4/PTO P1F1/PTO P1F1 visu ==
  note: 1) Add Subsystem or Model blocks as valid variant choices. 2) You cannot connect blocks at this level. At simulation, connectivity is automatically determined, based on the active variant and port name matching.
  Hydrodynamic Body : Subsystem  VariantControl=sv_b4_hydroBody
  Non-Hydro Body : Subsystem  VariantControl=sv_b4_nonHydroBody
  Conn : PMIOPort  Port=1  Side=Right

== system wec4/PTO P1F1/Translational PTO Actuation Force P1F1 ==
  Force : Inport
  Assignment{,1..3} (4 alike) : Assignment  IndexOptions=Index vector (dialog)  Indices=3  OutputSizes=1
  Bus Creator2 : BusCreator  Inputs=3
  Constant{,1..3} (4 alike) : Constant  Value=[0 0 0 0 0 0]
  InternalMechanics : Subsystem
  Mux : Mux  Inputs=2
  Mux1 : Mux  Inputs=2
  Mux2 : Mux  Inputs=8
  PS-Simulink Converter{,1..7} (8 alike) : nesl_utility/PS-Simulink Converter  PhysicalDomain=network_engine_domain  SubClassName=ps_output  LeftPortType=input  RightPortType=output  PseudoPeriodic=off  Frequencies=[]  Unit=1  AffineConversion=off
  Rigid Transform (Position) : sm_lib/Frames and Transforms/Rigid Transform  TranslationMethod=Cartesian  TranslationStandardOffset=0  TranslationLengthUnit=m  TranslationStandardAxis=+Z  TranslationCartesianOffset=pto.initDisp.initLinDisp + pto.loc  TranslationROffset=0  TranslationROffsetUnits=m  TranslationZOffset=0  TranslationZOffsetUnits=m  TranslationThetaOffset=0  TranslationThetaOffsetUnits=deg  RotationMethod=None  RotationAngleUnits=rad  RotationStandardAxis=+Y  RotationAngle=0  RotationArbitraryAxis=[0 1 0]  FollAlignAxisA=+X  BaseAlignAxisA=+Y  FollAlignAxisB=+Y  BaseAlignAxisB=+Z  RotationSequenceAxes=FollowerAxes  RotationSequence=XYX  RotationSequenceAngles=[0 0 0]  RotationSequenceAnglesUnits=deg  RotationMatrix=[1 0 0; 0 1 0; 0 0 1]
  Rigid Transform (Position)1 : sm_lib/Frames and Transforms/Rigid Transform  TranslationMethod=Cartesian  TranslationStandardOffset=0  TranslationLengthUnit=m  TranslationStandardAxis=+Z  TranslationCartesianOffset=pto.initDisp.initLinDisp + pto.loc  TranslationROffset=0  TranslationROffsetUnits=m  TranslationZOffset=0  TranslationZOffsetUnits=m  TranslationThetaOffset=0  TranslationThetaOffsetUnits=deg  RotationMethod=None  RotationAngleUnits=rad  RotationStandardAxis=+Y  RotationAngle=0  RotationArbitraryAxis=[0 1 0]  FollAlignAxisA=+X  BaseAlignAxisA=+Y  FollAlignAxisB=+Y  BaseAlignAxisB=+Z  RotationSequenceAxes=FollowerAxes  RotationSequence=XYX  RotationSequenceAngles=[0 0 0]  RotationSequenceAnglesUnits=deg  RotationMatrix=[1 0 0; 0 1 0; 0 0 1]
  Rigid Transform (Orientation) : sm_lib/Frames and Transforms/Rigid Transform  TranslationMethod=None  TranslationStandardOffset=0  TranslationLengthUnit=m  TranslationStandardAxis=+Z  TranslationCartesianOffset=0  TranslationROffset=0  TranslationROffsetUnits=m  TranslationZOffset=0  TranslationZOffsetUnits=m  TranslationThetaOffset=0  TranslationThetaOffsetUnits=deg  RotationMethod=RotationMatrix  RotationAngleUnits=rad  RotationStandardAxis=+Y  RotationAngle=0  RotationArbitraryAxis=[0 1 0]  FollAlignAxisA=+X  BaseAlignAxisA=+Y  FollAlignAxisB=+Y  BaseAlignAxisB=+Z  RotationSequenceAxes=FollowerAxes  RotationSequence=XYX  RotationSequenceAngles=[0 0 0]  RotationSequenceAnglesUnits=deg  RotationMatrix=pto.orientation.rotationMatrix
  Rigid Transform (Orientation)1 : sm_lib/Frames and Transforms/Rigid Transform  TranslationMethod=None  TranslationStandardOffset=0  TranslationLengthUnit=m  TranslationStandardAxis=+Z  TranslationCartesianOffset=0  TranslationROffset=0  TranslationROffsetUnits=m  TranslationZOffset=0  TranslationZOffsetUnits=m  TranslationThetaOffset=0  TranslationThetaOffsetUnits=deg  RotationMethod=RotationMatrix  RotationAngleUnits=rad  RotationStandardAxis=+Y  RotationAngle=0  RotationArbitraryAxis=[0 1 0]  FollAlignAxisA=+X  BaseAlignAxisA=+Y  FollAlignAxisB=+Y  BaseAlignAxisB=+Z  RotationSequenceAxes=FollowerAxes  RotationSequence=XYX  RotationSequenceAngles=[0 0 0]  RotationSequenceAnglesUnits=deg  RotationMatrix=pto.orientation.rotationMatrix
  Simulink-PS Converter : nesl_utility/Simulink-PS Converter  PhysicalDomain=network_engine_domain  SubClassName=ps_input  LeftPortType=input  RightPortType=output  PseudoPeriodic=off  Frequencies=[]  NoiseDistribution=none  NoiseParameters=[]  Unit=1  AffineConversion=off  InputFiltering=off  SimscapeFilterOrder=1  InputFilterTimeConstant=0.001  UdotUserProvided=1
  Translational PCC (Prismatic Joint) : sm_lib/Joints/Prismatic Joint  SenseConstraintForce=on  SenseConstraintForceX=off  SenseConstraintForceY=off  SenseConstraintForceZ=off  SenseConstraintTorque=on  SenseConstraintTorqueX=off  SenseConstraintTorqueY=off  SenseConstraintTorqueZ=off  SenseTotalForce=on  SenseTotalForceX=off  SenseTotalForceY=off  SenseTotalForceZ=off  SenseTotalTorque=on  SenseTotalTorqueX=off  SenseTotalTorqueY=off  SenseTotalTorqueZ=off  CompositeWrenchDir=BaseOnFollower  CompositeWrenchFrame=BaseFrame  EquilibriumPosition=0  EquilibriumPositionUnits=m  SpringStiffness=pto.k  SpringStiffnessUnits=N/m  DampingCoefficient=pto.c  DampingCoefficientUnits=N/(m/s)  TorqueActuationMode=InputTorque  MotionActuationMode=ComputedMotion  SensePosition=on  SenseVelocity=on  SenseAcceleration=on  SenseTorqueForce=on  PositionTargetSpecify=off  PositionTargetPriority=High  PositionTargetValue=0  PositionTargetValueUnits=m  VelocityTargetSpecify=off  VelocityTargetPriority=High  VelocityTargetValue=0  VelocityTargetValueUnits=m/s
  output : ToWorkspace  VariableName=pto1_out  SaveFormat=Structure With Time  SampleTime=-1
  F : PMIOPort  Port=1  Side=Right
  B : PMIOPort  Port=2  Side=Left
  Response : Outport
  ptoForce : Outport  Port=2
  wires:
  Bus Creator2/1 -> Response/1
  Assignment/1 -> Mux2/1, Bus Creator2/1, InternalMechanics/1(Position)  "position"
  Assignment1/1 -> Mux2/2, Bus Creator2/2, InternalMechanics/2(Velocity)  "velocity"
  Assignment2/1 -> Mux2/3, Bus Creator2/3  "acceleration"
  Force/1 -> Simulink-PS Converter/1
  Mux2/1 -> output/1
  Mux/1 -> Mux2/6  "forceConstraint"
  Mux1/1 -> Mux2/4  "forceTotal"
  PS-Simulink Converter4/1 -> Mux/1
  PS-Simulink Converter5/1 -> Mux/2
  PS-Simulink Converter6/1 -> Mux1/1
  PS-Simulink Converter7/1 -> Mux1/2
  Assignment3/1 -> ptoForce/1, Mux2/5  "forceActuation"
  Constant/1 -> Assignment/1
  PS-Simulink Converter/1 -> Assignment/2
  Constant1/1 -> Assignment1/1
  PS-Simulink Converter1/1 -> Assignment1/2
  Constant2/1 -> Assignment2/1
  PS-Simulink Converter2/1 -> Assignment2/2
  InternalMechanics/1(Force) -> Mux2/7  "forceInternalMechanics"
  InternalMechanics/2(Power) -> Mux2/8  "powerInternalMechanics"
  Constant3/1 -> Assignment3/1
  PS-Simulink Converter3/1 -> Assignment3/2  "forceActuation"
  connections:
  Rigid Transform (Position)/RConn1 -- Rigid Transform (Orientation)/LConn1
  Rigid Transform (Position)1/RConn1 -- Rigid Transform (Orientation)1/LConn1
  Simulink-PS Converter/RConn1 -- Translational PCC (Prismatic Joint)/LConn2
  Rigid Transform (Orientation)/RConn1 -- Translational PCC (Prismatic Joint)/LConn1
  Rigid Transform (Position)/LConn1 -- B/RConn1
  Translational PCC (Prismatic Joint)/RConn5 -- PS-Simulink Converter3/LConn1
  Translational PCC (Prismatic Joint)/RConn9 -- PS-Simulink Converter7/LConn1
  Rigid Transform (Orientation)1/RConn1 -- Translational PCC (Prismatic Joint)/RConn1
  Translational PCC (Prismatic Joint)/RConn4 -- PS-Simulink Converter2/LConn1
  Translational PCC (Prismatic Joint)/RConn7 -- PS-Simulink Converter5/LConn1
  Translational PCC (Prismatic Joint)/RConn3 -- PS-Simulink Converter1/LConn1
  Rigid Transform (Position)1/LConn1 -- F/RConn1
  Translational PCC (Prismatic Joint)/RConn8 -- PS-Simulink Converter6/LConn1
  Translational PCC (Prismatic Joint)/RConn2 -- PS-Simulink Converter/LConn1
  Translational PCC (Prismatic Joint)/RConn6 -- PS-Simulink Converter4/LConn1

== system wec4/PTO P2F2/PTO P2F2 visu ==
  note: 1) Add Subsystem or Model blocks as valid variant choices. 2) You cannot connect blocks at this level. At simulation, connectivity is automatically determined, based on the active variant and port name matching.
  Hydrodynamic Body : Subsystem  VariantControl=sv_b5_hydroBody
  Non-Hydro Body : Subsystem  VariantControl=sv_b5_nonHydroBody
  Conn : PMIOPort  Port=1  Side=Right
